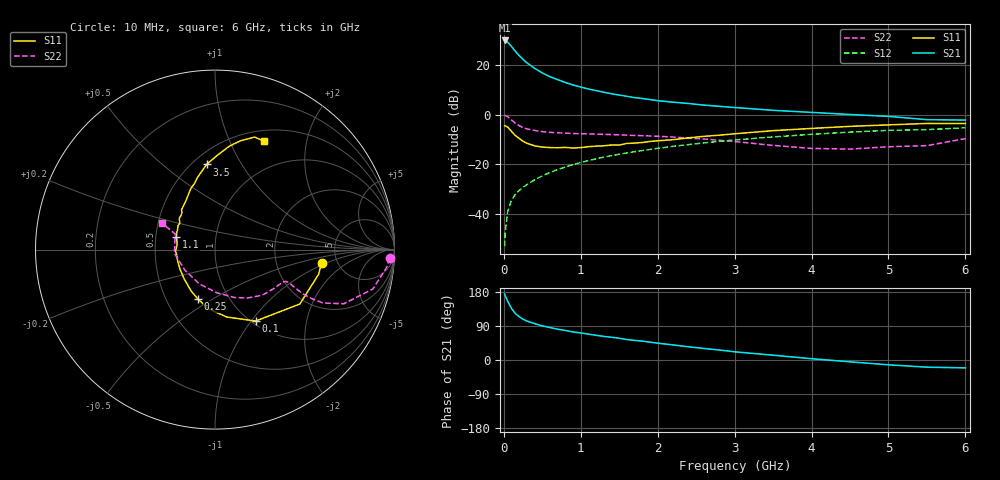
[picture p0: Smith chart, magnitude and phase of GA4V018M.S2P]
! Infineon Technologies  Discrete & RF Semiconductors
! BF775
! Si NPN RF Bipolar Junction Transistor in SOT23
! VCE = 4 V  IC = 18 mA
! Common Emitter S-Parameters:  May  1996
# GHz  S  MA  R  50
!  f  S11  S21  S12  S22
! GHz  MAG  ANG  MAG  ANG  MAG  ANG  MAG  ANG
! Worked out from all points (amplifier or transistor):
!   36 points, 10 MHz to 6 GHz, reference 50 ohm
!   highest |S21| = 29.7 dB at 10 MHz (marker M1)
!   |S21| within 3 dB of that: start of sweep to 114.8 MHz
!   unconditionally stable (mu >= 1): 428 MHz to 2.989 GHz
!   at 250 MHz: K = 0.84, MSG = 25.6 dB, |S12| = -29.2 dB
!   at 1.4 GHz: K = 1.11, MAG = 10.4 dB, |S12| = -16.5 dB
!   at 6 GHz: K = 0.94, MSG = 1.5 dB, |S12| = -5.3 dB
!   S11 on the Smith chart (normalised r, x): 10 MHz: 3.78, -0.85; 100 MHz: 1.04, -1.05; 250 MHz: 0.72, -0.43; 1.1 GHz: 0.64, +0.10; 3.5 GHz: 0.58, +0.72; 6 GHz: 0.63, +1.35
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0.01  0.5984 -6.9  30.67 174.4  0.0023 84.5  0.9741 -2.8
0.02  0.5933 -13.5  30.16 169.0  0.0046 80.5  0.961 -6.0
0.05  0.5613 -32.7  28.23 154.8  0.0115 77.3  0.9066 -14.0
0.1  0.4578 -60.4  23.18 135.9  0.0193 69.0  0.7785 -22.8
0.15  0.3813 -80.1  18.58 122.6  0.0253 65.8  0.6718 -26.3
0.2  0.3327 -95.9  15.24 114.1  0.0301 65.6  0.5995 -26.9
0.25  0.2915 -109.1  12.75 107.5  0.0348 65.7  0.5487 -26.7
0.3  0.2657 -120.2  10.91 102.8  0.0395 67.0  0.5183 -26.1
0.4  0.2362 -137.1  8.464 96.0  0.0494 67.9  0.48 -25.1
0.5  0.2235 -151.0  6.842 90.1  0.059 69.1  0.4568 -24.2
0.6  0.2179 -162.0  5.757 85.6  0.0691 69.5  0.4402 -24.1
0.8  0.22 -178.1  4.401 77.9  0.0894 69.2  0.4252 -25.0
0.9  0.2131 173.8  3.924 74.1  0.0994 68.7  0.4169 -25.5
1.1  0.2276 161.7  3.265 68.3  0.1198 67.8  0.4105 -28.1
1.3  0.2365 151.9  2.804 62.3  0.1403 66.1  0.4021 -30.3
1.6  0.2644 138.9  2.326 53.9  0.1703 63.4  0.3868 -35.4
2.2  0.3142 121.4  1.773 39.8  0.2309 57.1  0.3541 -46.8
3  0.4125 103.8  1.387 21.6  0.3102 47.6  0.2889 -67.6
3.5  0.4766 95.7  1.219 12.7  0.3568 41.1  0.2411 -87.5
4.5  0.5808 82.2  1.004 -4.8  0.4457 27.9  0.2031 -145.8
5.5  0.6647 70.6  0.792 -18.9  0.4997 12.9  0.2388 158.6
6  0.6627 65.7  0.776 -20.8  0.5444 8.8  0.3297 153.4
